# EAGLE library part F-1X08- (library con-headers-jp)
FEMALE HEADER
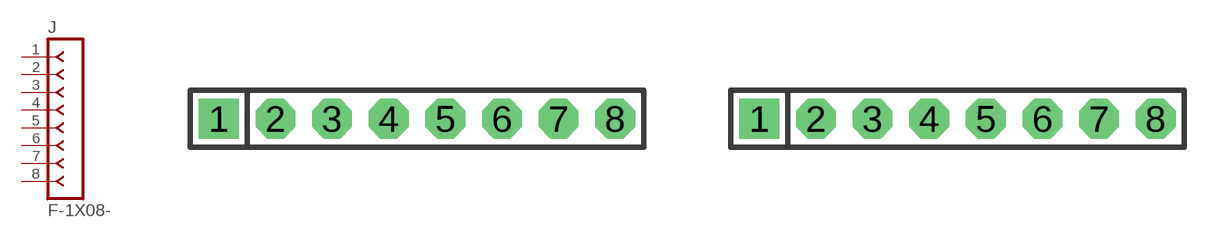
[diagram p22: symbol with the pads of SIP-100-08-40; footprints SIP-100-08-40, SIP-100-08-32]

Designator prefix J

## F-1X08-SIP-100-40  [SIP-100-08-40]
1  1  pas
2  2  pas
3  3  pas
4  4  pas
5  5  pas
6  6  pas
7  7  pas
8  8  pas

## F-1X08-SIP-100-32  [SIP-100-08-32]
Pads as for SIP-100-08-40

## F-1X08-SIP-100-32Y  [SIP-100-08-32Y]
Pads as for SIP-100-08-40

## F-1X08-SIP-100-40Y  [SIP-100-08-40Y]
Pads as for SIP-100-08-40

## F-1X08-KK-4455-B08  [KK-4455-B08]
Pads as for SIP-100-08-40

## F-1X08-KK-4455-C08  [KK-4455-C08]
Pads as for SIP-100-08-40

## F-1X08-KK-4455-A08  [KK-4455-A08]
Pads as for SIP-100-08-40

## Footprint SIP-100-08-40 (pad centres in mm)
SIP Header - 0.1", 40 mil drill
drill 1.016 pad 1.778 square: 1 -8.89,0
drill 1.016 pad 1.778 octagon: 2 -6.35,0; 3 -3.81,0; 4 -1.27,0; 5 1.27,0; 6 3.81,0; 7 6.35,0; 8 8.89,0

## Footprint SIP-100-08-32 (pad centres in mm)
SIP Header - 0.1", 32 mil drill
drill 0.813 pad 1.778 square: 1 -8.89,0
drill 0.813 pad 1.778 octagon: 2 -6.35,0; 3 -3.81,0; 4 -1.27,0; 5 1.27,0; 6 3.81,0; 7 6.35,0; 8 8.89,0

## Footprint SIP-100-08-32Y (pad centres in mm)
SIP Header - 0.1", 32 mil drill
drill 0.813 long: 1 -8.89,0; 2 -6.35,0; 3 -3.81,0; 4 -1.27,0; 5 1.27,0; 6 3.81,0; 7 6.35,0; 8 8.89,0

## Footprint SIP-100-08-40Y (pad centres in mm)
SIP Header - 0.1", 40 mil drill
drill 1.016 long: 1 -8.89,0; 2 -6.35,0; 3 -3.81,0; 4 -1.27,0; 5 1.27,0; 6 3.81,0; 7 6.35,0; 8 8.89,0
